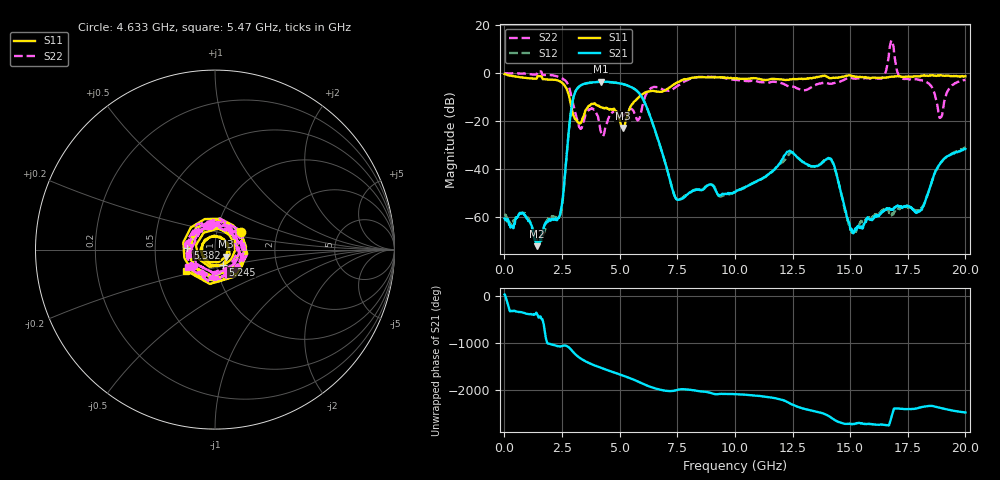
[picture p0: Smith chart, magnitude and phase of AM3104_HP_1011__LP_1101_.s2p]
!Created with skrf (http://scikit-rf.org).
# Hz S RI R 50.0
!freq ReS11 ImS11 ReS21 ImS21 ReS12 ImS12 ReS22 ImS22
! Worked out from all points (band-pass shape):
!   1601 points, 10 MHz to 20 GHz, reference 50 ohm
!   highest |S21| = -3.53 dB at 4.183 GHz (marker M1); lowest = -72.1 dB at 1.409 GHz (marker M2)
!   |S21| within 3 dB of the highest: 3.154 GHz to 5.636 GHz (2.481 GHz wide, 56.5 % of centre)
!   lowest |S11| = -22.8 dB at 5.132 GHz (marker M3), VSWR 1.16, Z = 56.2 - j4.49 ohm
!   |S11| at or under -10 dB: 2.815 GHz to 5.83 GHz (3.015 GHz wide, 69.8 % of centre)
!   |S22| runs from -26.3 to 13.6 dB; largest |S21 - S12| = 0.07
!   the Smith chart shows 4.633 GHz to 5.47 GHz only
!   S11 on the Smith chart (normalised r, x): 4.633 GHz: 1.31, +0.27; 5.245 GHz: 1.07, -0.18; 5.382 GHz: 0.73, +0.02; 5.47 GHz: 0.71, -0.17
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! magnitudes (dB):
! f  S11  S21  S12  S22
! 10 MHz  -0.4  -60.6  -58.9  0.0
! 1.409 GHz  -2.1  -72.1  -70.2  -0.1
! 2.421 GHz  -3.5  -58.6  -59.3  -1.8
! 2.934 GHz  -15.5  -13.1  -13.1  -10.9
! 3.346 GHz  -20.3  -4.9  -5.0  -22.9
! 4.183 GHz  -14.2  -3.5  -3.6  -24.4
! 4.633 GHz  -15.2  -3.7  -3.8  -17.1
! 5.132 GHz  -22.8  -4.5  -4.6  -17.9
! 5.245 GHz  -20.6  -4.8  -4.8  -16.7
! 5.382 GHz  -16.2  -5.3  -5.3  -15.4
! 5.47 GHz  -14.0  -5.6  -5.7  -14.9
! 6.682 GHz  -7.7  -28.1  -28.1  -5.9
! 7.506 GHz  -3.9  -52.8  -52.8  -5.4
! 10.01 GHz  -2.3  -49.7  -49.5  -2.9
! 12.33 GHz  -2.8  -32.7  -34.1  -5.6
! 13.34 GHz  -2.1  -38.9  -39.0  -5.8
! 14.22 GHz  -2.1  -36.7  -36.9  -4.3
! 15.1 GHz  -1.3  -66.2  -65.8  -2.2
! 16.68 GHz  -1.6  -56.6  -57.7  7.3
! 18.04 GHz  -1.4  -57.5  -56.4  -2.9
! 18.91 GHz  -0.8  -37.6  -37.7  -18.6
! 20 GHz  -1.3  -31.6  -31.0  -2.8
